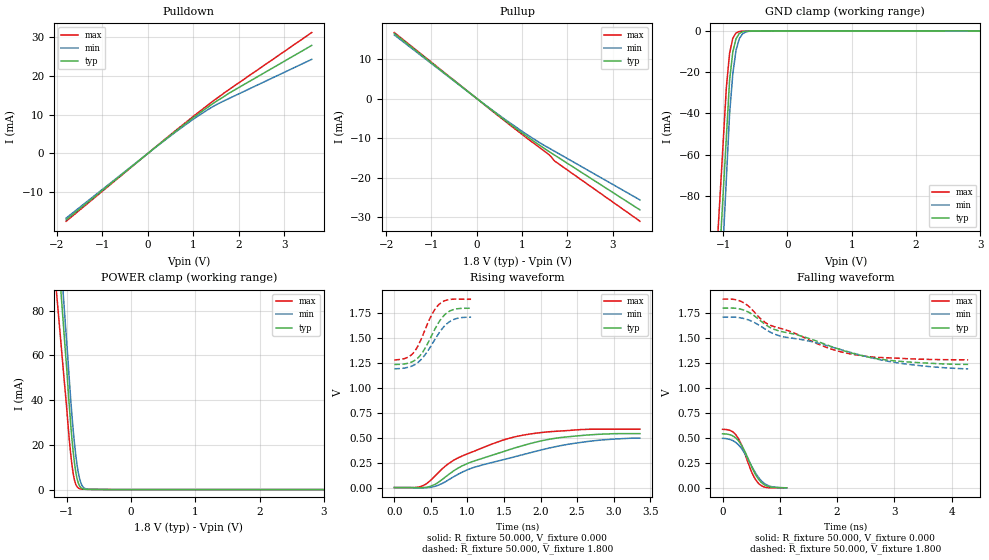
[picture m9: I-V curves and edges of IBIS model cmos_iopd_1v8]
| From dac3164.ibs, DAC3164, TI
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[Model]   cmos_iopd_1v8
Model_type I/O
Vinl=4.500E-01
Vinh=1.080E+00
Vref=0.000E+00
Rref=1.000E+06
Cref=0.000E+00
Vmeas=9.000E-01
C_comp   1.070E-12   1.070E-12   1.070E-12
[Voltage Range]   1.800E+00   1.710E+00   1.890E+00
[POWER Clamp Reference]   1.800E+00   1.710E+00   1.890E+00
[GND Clamp Reference]   0.000E+00   0.000E+00   0.000E+00
[Pullup Reference]   1.800E+00   1.710E+00   1.890E+00
[Pulldown Reference]   0.000E+00   0.000E+00   0.000E+00
[Temperature Range]   25   85   -40
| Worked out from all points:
|   slope of the pulldown table from 0 to 0.27 V, typ, clamps not added: 105 ohm
|   slope of the pullup table from 0 to 0.27 V, typ, clamps not added: 112 ohm
|   GND clamp passes 1 mA (typ) near -0.73 V on its own axis
|   POWER clamp passes 1 mA (typ) near -0.78 V on its own axis
|   rising waveform, R_fixture 50.000, V_fixture 0.000: 20-80 % time 1.11ns typ, 1.33ns min, 899ps max; typ from 0.001 V to 0.542 V
|   falling waveform, R_fixture 50.000, V_fixture 0.000: 20-80 % time 278ps typ, 307ps min, 244ps max; typ from 0.542 V to 0.001 V
|   rising waveform, R_fixture 50.000, V_fixture 1.800: 20-80 % time 257ps typ, 289ps min, 229ps max; typ from 1.24 V to 1.8 V
|   falling waveform, R_fixture 50.000, V_fixture 1.800: 20-80 % time 1.63ns typ, 1.95ns min, 1.29ns max; typ from 1.8 V to 1.24 V
[GND Clamp]
-1.8V     -518.4mA   -605mA     -482.8mA
-950mV    -51.38mA   -71.58mA   -27.3mA
-900mV    -23.91mA   -40.2mA    -10.85mA
-850mV    -10.2mA    -20.83mA   -3.517mA
-800mV    -3.824mA   -9.382mA   -1.017mA
-750mV    -1.288mA   -3.836mA   -302.4uA
-700mV    -411.3uA   -1.472mA   -137.1uA
-600mV    -138.8uA   -193.7uA   -104uA
3.6V      23.98uA    36.49uA    15.85uA
[Power Clamp]
-1.8V     365.2mA    387.4mA    299.8mA
-1.74V    341.9mA    362mA      279.1mA
-1.06V    77.11mA    89.83mA    55.91mA
-1.04V    69.32mA    81.84mA    49.26mA
-960mV    37.66mA    49.43mA    22.5mA
-920mV    23.15mA    33.79mA    11.41mA
-880mV    12.09mA    20.93mA    4.368mA
-860mV    8.053mA    15.67mA    2.442mA
-820mV    2.958mA    7.657mA    712.3uA
-760mV    495.2uA    1.737mA    212.6uA
-640mV    81.27uA    116.2uA    112.4uA
3.6V      0A         0A         0A
[Pullup]
-1.82V    16.44mA    16.09mA    16.7mA
40mV      -364.6uA   -352.9uA   -377.6uA
1.02V     -8.884mA   -8.464mA   -9.256mA
1.58V     -13.33mA   -12.46mA   -14.08mA
1.72V     -14.34mA   -13.37mA   -15.84mA
3.6V      -28.18mA   -25.68mA   -31.07mA
[Pulldown]
-1.8V     -17.17mA   -16.72mA   -17.54mA
580mV     5.467mA    5.277mA    5.626mA
1.28V     11.63mA    11.02mA    12.14mA
1.48V     13.27mA    12.43mA    13.94mA
1.78V     15.53mA    14.17mA    16.47mA
3.6V      27.88mA    24.28mA    31.2mA
[Rising Waveform]
R_fixture = 50.000
V_fixture = 0.000
V_fixture_min = 0.000
V_fixture_max = 0.000
|  time   V(typ)   V(min)   V(max)
0s        904.3uV    782.5uV    597.2uV
330ps     -1.011mV   -2.075mV   5.855mV
490ps     12.55mV    3.241mV    69.71mV
710ps     113.1mV    64.13mV    223.4mV
850ps     186.5mV    125mV      290.4mV
1.08ns    264.5mV    201.3mV    362mV
1.65ns    398.8mV    310.3mV    510.2mV
2.28ns    503mV      422mV      568.5mV
2.78ns    534.6mV    474.4mV    586.2mV
3.36ns    541.6mV    496.2mV    586.2mV
[Falling Waveform]
R_fixture = 50.000
V_fixture = 0.000
V_fixture_min = 0.000
V_fixture_max = 0.000
|  time   V(typ)   V(min)   V(max)
0s        541.6mV    496.2mV    586.2mV
150ps     527.9mV    480.5mV    570.1mV
250ps     489.6mV    445.8mV    517.2mV
360ps     397.7mV    369.9mV    388.2mV
520ps     196.8mV    204.6mV    144mV
580ps     129.7mV    145.2mV    80.27mV
640ps     78.15mV    95.64mV    38.61mV
720ps     35.18mV    49.03mV    10.8mV
820ps     10.91mV    18.36mV    982.3uV
1.12ns    904.3uV    782.5uV    597.2uV
[Rising Waveform]
R_fixture = 50.000
V_fixture = 1.800
V_fixture_min = 1.710
V_fixture_max = 1.890
|  time   V(typ)   V(min)   V(max)
0s        1.237V     1.192V     1.282V
160ps     1.244V     1.203V     1.3V
270ps     1.273V     1.231V     1.361V
330ps     1.307V     1.26V      1.432V
400ps     1.374V     1.314V     1.548V
520ps     1.54V      1.444V     1.746V
630ps     1.683V     1.571V     1.85V
710ps     1.748V     1.639V     1.881V
810ps     1.787V     1.686V     1.891V
1.05ns    1.8V       1.71V      1.89V
[Falling Waveform]
R_fixture = 50.000
V_fixture = 1.800
V_fixture_min = 1.710
V_fixture_max = 1.890
|  time   V(typ)   V(min)   V(max)
0s        1.8V       1.71V      1.89V
330ps     1.787V     1.701V     1.865V
510ps     1.741V     1.669V     1.789V
670ps     1.67V      1.617V     1.69V
800ps     1.615V     1.57V      1.637V
1.01ns    1.568V     1.52V      1.597V
1.39ns    1.518V     1.484V     1.515V
2.08ns    1.38V      1.382V     1.36V
2.87ns    1.28V      1.27V      1.303V
4.29ns    1.237V     1.192V     1.282V
[Ramp]
dV/dt_r   3.2417E-01/1.1109E-09   2.9794E-01/1.3271E-09   3.5095E-01/8.9375E-10
dV/dt_f   3.3800E-01/1.6255E-09   3.1047E-01/1.9505E-09   3.6473E-01/1.2864E-09
R_load = 50
